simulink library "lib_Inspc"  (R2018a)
settings: Solver=ode3  StartTime=0.0  StopTime=1  FixedStep=0.02/16384  RelTol=1e-3
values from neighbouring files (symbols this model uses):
  Tstep = 0.0001    [TestInspcStimuli_init.m]
undefined symbols (not defined in the file or in its folder): stimuli_path

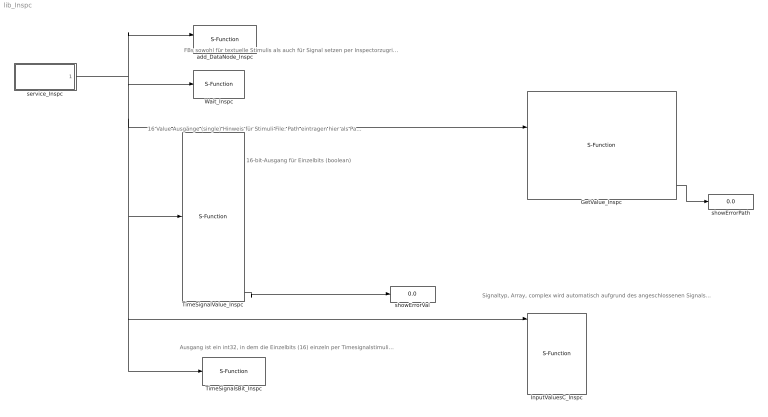
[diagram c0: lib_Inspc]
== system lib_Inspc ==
  note: Ausgang ist ein int32, in dem die Einzelbits (16) einzeln per Timesignalstimuli oder inspector belegt werden können. Parameter Name: Namen der Einzelbits. Werte in Timesignal-File: ==0 ist 0, !=0 setzt das Bit.
  note: Signaltyp, Array, complex wird automatisch aufgrund des angeschlossenen Signals erkannt. Es gibt teils Probleme mit back-probagation, wenn Simulink die Anzahl ArrayElemente nicht festlegen kann. Man muss dieses Problem lösen, indem die Leitung eindeutig bestimmt wird beispielsweise an den Ports. Hier kann man das Signal leider nicht bestimmen. . Sonderfunktion: Wenn Name mit * beginnt, dann muss der Eingang ein Pointer-Alias-Typ sein. Dann wird dessen Inhalt dargestellt.
  note: 16 Value-Ausgänge (single) Hinweis für Stimuli-File: Path eintragen hier als Parameter. Das File kann ein m-File sein, insbesondere für parametersetzen. Die TimeSignals-Stimuli sind als Kommentar eingetragen, in der Form: %time:0.5: Signal=0.5, Signal2 = 0.7; Keyword ist "%time:" * Zeilen ohne diess Keyword werden ignoriert - andere m-Script-Befehle. * Mehr als ein Signal zur gleichen Zeit möglich. Trennung mit Komma * Zeiten können im Stimuli-File durcheinander sein, werden sortiert. Parameter, Konfiguration der Signalnamen: ' Name in Reflection tree' Erscheint in Reflection-Baum und im Symbol, ** muss für das Modell eindeutig sein ** kann auch über Stringvariable vermittelt werden, insbesondere für Einsatz in Lib-Modulen. * 'name 1..12' ** '2:name': Array von 2 Elementen, 1..6 möglich, since 2015-011-24 ** 'C:name': complex float output, derzeit noch nicht unterstützt ** 'C2:name': complex vector, derzeit noch nicht unterstützt Datentyp ist ausschließlich float. Letzter Ausgang ist error, 0: Kein Fehler,
  note: 16-bit-Ausgang für Einzelbits (boolean)
  note: FBs sowohl für textuelle Stimulis als auch für Signal setzen per Inspectorzugriff (Reflection).
  GetValue_Inspc : S-Function  FunctionName=get_GetValue_Inspc_SfH  Parameters=Tstep, path1, path2, path3, path4, path5, path6  SFunctionDeploymentMode=off  EnableBusSupport=off  mask{Tstep=Tstep, path1='path.to.variable', path2='path.to.variable', path3='path.to.variable', path4='path.to.variable', path5='path.to.variable', path6='path.to.variable'}
      mask help: Accesses any data via Reflection. @param Tstep: It accesses data and bring to output in this step time. @param: Reflection-Path to access data @Input1: handle of Service_Inspc @Input2: control input. If not 0, it initializes the addresses with given paths. It is especially from Output of add_DataNode_Inspc. Only if this FB has added the node, it should init. @Output 1..6: Shows the values. @Output 7: Debug, should be 0, elsewhere path mismatch.
  InputValuesC_Inspc : S-Function  FunctionName=step_InputValues_Inspc_SfH  Parameters=nameRefl n1 n2 n3 n4 n5 n6 n7 n8 n9 n10 n11 n12  SFunctionDeploymentMode=off  EnableBusSupport=off  mask{nameRefl='NameStruct', n1='X1', n2='X2', n3='X3', n4='X4', n5='X5', n6='X6', n7='X7', n8='X8', n9='X9', n10='X10', n11='X11', n12='X12'}
      mask prompts: nameRefl "Name in reflection-tree"; n1 "name 1"; n2 "name 2"; n3 "name 3"; n4 "name 4"; n5 "name 5"; n6 "name 6"; n7 "name 7"; n8 "name 8"; n9 "name 9"; n10 "name 10"; n11 "name 11"; n12 "name 12"
  TimeSignalValue_Inspc : S-Function  Description=|  FunctionName=values_TimeSignals_Inspc_SfH  Parameters=Tstep filepath nameRefl nrofStimuli n1 n2 n3 n4 n5 n6 n7 n8 n9 n10 n11 n12 n13 n14 n15 n16  SFunctionDeploymentMode=off  EnableBusSupport=off  mask{Tstep=Tstep, filepath=stimuli_path, nameRefl='TimeSignals_1', nrofStimuli=25, n1='signal1', n2='signal2', n3='', n4='', n5='', n6='', n7='', n8='', n9='', n10='', n11='', n12='', n13='', n14='', n15='', n16=''}
      | A combined stimuli and inspector function block.
      | Stimuli file path: file contains stimuli in form:
      |   %time:0: stimuli.namex = 5000.0, stimuli.namey = 50.0 -10; 
      | Name in reflection-tree: Name of this function block for stimuli and inspector access
      | name1..12: output type and name, base type is single always.
      | C2:namexy  A complex array of 2 elements
      | 6:namexy An array of 6 elements (max).
      | C:namexy  A 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
      mask prompts: filepath "Stimuli file path"; nameRefl "Name in reflection-tree"; nrofStimuli "max number of stimuli entries"; n1 "name 1"; n2 "name 2"; n3 "name 3"; n4 "name 4"; n5 "name 5"; n6 "name 6"; n7 "name 7"; n8 "name 8"; n9 "name 9"; n10 "name 10"; n11 "name 11"; n12 "name 12"; n13 "name 13"; n14 "name 14"; n15 "name 15"; n16 "name 16"
      mask help: A combined stimuli and inspector function block. Stimuli file path: file contains stimuli in form: %time:0: stimuli.namex = 5000.0, stimuli.namey = 50.0 -10; Name in reflection-tree: Name of this function block for stimuli and inspector access name1..12: output type and name, base type is single always. C2:namexy A complex array of 2 elements 6:namexy An array of 6 elements (max). C:namexy A complex single namexy A real single.
  TimeSignalsBit_Inspc : S-Function  FunctionName=TimeSignalsBit_Inspc_mex  Parameters=filepath nameRefl nrofStimuli n1 n2 n3 n4 n5 n6 n7 n8 n9 n10 n11 n12 n13 n14 n15 n16  SFunctionDeploymentMode=off  EnableBusSupport=off  mask{filepath=stimuli_path, nameRefl='BinarySignals', nrofStimuli=25, n1='bit0', n2='bit1', n3='', n4='', n5='', n6='', n7='', n8='', n9='', n10='', n11='', n12='', n13='', n14='', n15='', n16=''}
      mask prompts: filepath "Stimuli file path"; nameRefl "Name in reflection tree"; nrofStimuli "max number of stimuli entries"; n1 "name 1"; n2 "name 2"; n3 "name 3"; n4 "name 4"; n5 "name 5"; n6 "name 6"; n7 "name 7"; n8 "name 8"; n9 "name 9"; n10 "name 10"; n11 "name 11"; n12 "name 12"; n13 "name 13"; n14 "name 14"; n15 "name 15"; n16 "name 16"
  Wait_Inspc : S-Function  FunctionName=step_Wait_Inspc_SfH  Parameters=Tstep cyclesStart delay_ms  SFunctionDeploymentMode=off  EnableBusSupport=off  mask{Tstep=Tstep, cyclesStart=20, delay_ms=0}
      mask prompts: cyclesStart "cycles-start"; delay_ms "delay [ms]"
  add_DataNode_Inspc : S-Function  FunctionName=addObj_DataNode_Inspc_SfH  Parameters=name1Refl name2Refl  SFunctionDeploymentMode=off  EnableBusSupport=off  mask{name1Refl='main', name2Refl='_data'}
      mask prompts: name1Refl "Name in reflection tree"; name2Refl "Name part2, concatenated"
      mask help: Registers a Object-FB as a node for reflection access. Usual there is a special Object-FB which presents a bus of signals and some more Object-FB references. That ones output should be used. Because this FB is connected to handle outputs it is calculated in the Tinit time. @Input1: handle of Service_Inspc: connect Output 1 from Service_Inspc. @Input2: handle of any Object-FB. The Object-FB should have refelction information. @param name1_param first part of the name. The 2 parts of name offers the capability to use a instance name given in a variable and a constant part of name for this block.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
  service_Inspc : Subsystem  mask{Tstep=Tstep, IpPort='UDP:0.0.0.0:60094'}
  showErrorPath : Display
  showErrorVal : Display
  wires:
  service_Inspc/1(Out1) -> add_DataNode_Inspc/1, InputValuesC_Inspc/1, TimeSignalsBit_Inspc/1, TimeSignalValue_Inspc/1, GetValue_Inspc/1, Wait_Inspc/1
  GetValue_Inspc/7 -> showErrorPath/1
  TimeSignalValue_Inspc/17 -> showErrorVal/1

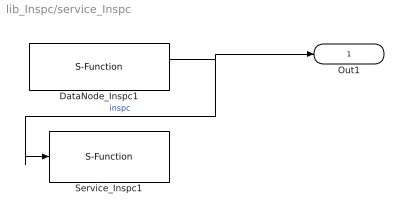
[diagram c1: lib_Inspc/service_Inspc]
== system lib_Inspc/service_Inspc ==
  DataNode_Inspc1 : S-Function  FunctionName=create_DataNode_Inspc_SfH  Parameters=50, Tstep  SFunctionDeploymentMode=off  EnableBusSupport=off
  Service_Inspc1 : S-Function  FunctionName=step_Service_Inspc_SfH  Parameters=Tstep, IpPort  SFunctionDeploymentMode=off  EnableBusSupport=off
  Out1 : Outport  OutDataTypeStr=uint32  PortDimensions=1
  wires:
  DataNode_Inspc1/1 -> Service_Inspc1/1, Out1/1  "inspc"
